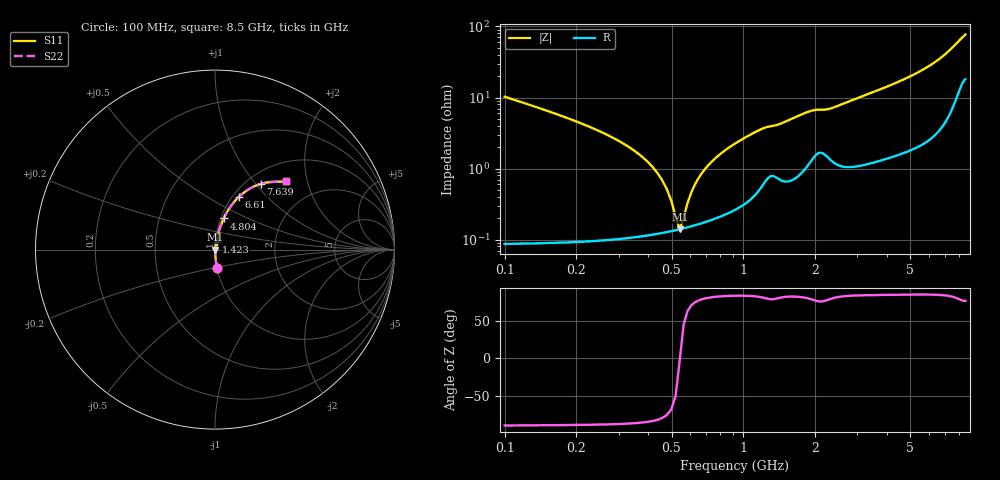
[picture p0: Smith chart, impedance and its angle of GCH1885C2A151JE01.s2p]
!Murata Part Number: GCH1885C2A151JE01
!These Parameters are Measured in Series Mode Connection
!Data Generated on Jun 19, 2026
!  o--ll--o
!Port1  Port2
!  o------o
!Operation Temp=25[degC], DC Bias Voltage=0[V]
!Freq. Start=100[MHz] Stop=9[GHz] 401[Steps]
# Hz S RI R 50
!Freq.(Hz) S11(Real) S11(Imag) S21(Real) S21(Imag) S12(Real) S12(Imag) S22(Real) S22(Imag)
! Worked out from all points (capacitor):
!   401 points, 100 MHz to 8.5 GHz, reference 50 ohm
!   read as one part in series: C = 150 pF near 142 MHz
!   lowest |Z| = 140 mohm at 541 MHz (marker M1)
!   series resonance near 541.9 MHz, so ESL is about 580 pH
!   S11 on the Smith chart (normalised r, x): 100 MHz: 1.00, -0.21; 1.423 GHz: 1.01, +0.08; 4.804 GHz: 1.03, +0.37; 6.61 GHz: 1.07, +0.69; 7.639 GHz: 1.16, +1.07; 8.5 GHz: 1.36, +1.50
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1e8  0.0112 -0.1013  0.9888 0.1013  0.9888 0.1013  0.0112 -0.1013
3.94e8  0.0013 -0.0127  0.9987 0.0127  0.9987 0.0127  0.0013 -0.0127
4.57e8  0.00128 -0.00671  0.9987 0.00671  0.9987 0.00671  0.00128 -0.00671
5.2e8  0.00135 -0.00162  0.9986 0.00162  0.9986 0.00162  0.00135 -0.00162
5.41e8  0.00139 -6.66e-05  0.9986 6.66e-05  0.9986 6.66e-05  0.00139 -6.66e-05
5.62e8  0.00144 0.00143  0.9986 -0.00143  0.9986 -0.00143  0.00144 0.00143
5.83e8  0.00149 0.00287  0.9985 -0.00287  0.9985 -0.00287  0.00149 0.00287
6.25e8  0.00161 0.00563  0.9984 -0.00563  0.9984 -0.00563  0.00161 0.00563
6.67e8  0.00176 0.00824  0.9982 -0.00824  0.9982 -0.00824  0.00176 0.00824
8.14e8  0.00242 0.0166  0.9976 -0.0166  0.9976 -0.0166  0.00242 0.0166
1.129e9  0.00541 0.0324  0.9946 -0.0324  0.9946 -0.0324  0.00541 0.0324
1.423e9  0.0086 0.0412  0.9914 -0.0412  0.9914 -0.0412  0.0086 0.0412
1.507e9  0.00854 0.045  0.9915 -0.045  0.9915 -0.045  0.00854 0.045
1.906e9  0.016 0.0615  0.984 -0.0615  0.984 -0.0615  0.016 0.0615
2.914e9  0.0189 0.0909  0.9811 -0.0909  0.9811 -0.0909  0.0189 0.0909
4.3e9  0.0378 0.1491  0.9622 -0.1491  0.9622 -0.1491  0.0378 0.1491
4.804e9  0.0485 0.1739  0.9515 -0.1739  0.9515 -0.1739  0.0485 0.1739
5.707e9  0.0776 0.2264  0.9224 -0.2264  0.9224 -0.2264  0.0776 0.2264
6.61e9  0.1311 0.2918  0.8689 -0.2918  0.8689 -0.2918  0.1311 0.2918
7.114e9  0.181 0.3317  0.819 -0.3317  0.819 -0.3317  0.181 0.3317
7.639e9  0.2559 0.3664  0.7441 -0.3664  0.7441 -0.3664  0.2559 0.3664
8.5e9  0.3965 0.3834  0.6035 -0.3834  0.6035 -0.3834  0.3965 0.3834
